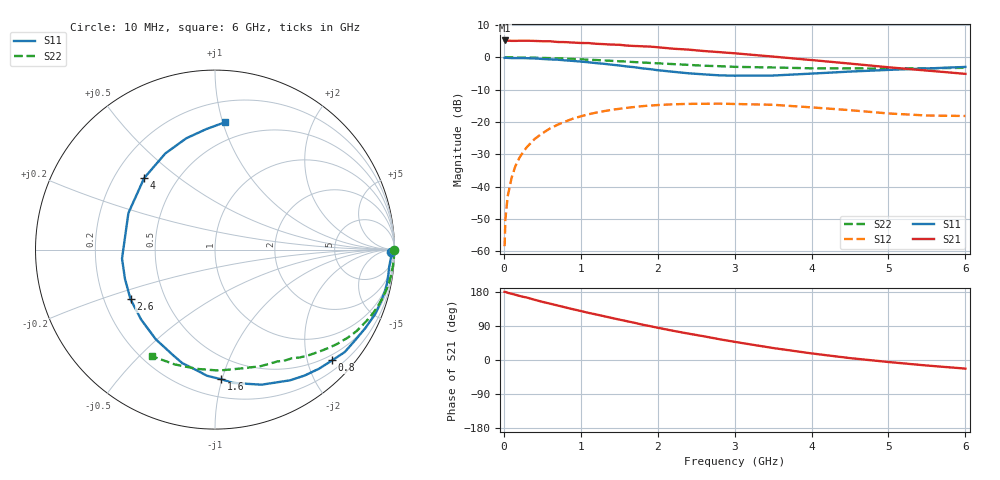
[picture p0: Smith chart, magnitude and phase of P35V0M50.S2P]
! SIEMENS Small Signal Semiconductors
! BFP181
! Si NPN RF Bipolar Junction Transistor in SOT143
! VCE = 5 V  IC = 0.5 mA
! Common Emitter S-Parameters:  March  1996
# GHz  S  MA  R  50
!  f  S11  S21  S12  S22
! GHz  MAG  ANG  MAG  ANG  MAG  ANG  MAG  ANG
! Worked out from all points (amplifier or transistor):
!   36 points, 10 MHz to 6 GHz, reference 50 ohm
!   highest |S21| = 5.2 dB at 10 MHz (marker M1)
!   |S21| within 3 dB of that: start of sweep to 2.476 GHz
!   unconditionally stable (mu >= 1): 3.793 GHz to end of sweep
!   at 250 MHz: K = 0.07, MSG = 17.2 dB, |S12| = -29.3 dB
!   at 1.4 GHz: K = 0.42, MSG = 10.1 dB, |S12| = -16.2 dB
!   at 6 GHz: K = 1.42, MAG = 2.6 dB, |S12| = -18.1 dB
!   S11 on the Smith chart (normalised r, x): 10 MHz: 69, -53; 800 MHz: 0.39, -2.46; 1.6 GHz: 0.33, -0.99; 2.6 GHz: 0.31, -0.25; 4 GHz: 0.33, +0.38; 6 GHz: 0.35, +1.02
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0.01  0.982 -0.8  1.827 179.8  0.0012 82.2  0.9999 -0.2
0.02  0.986 -1.2  1.825 179.7  0.0031 82.1  0.9998 -0.5
0.05  0.9817 -2.5  1.817 177.4  0.0071 91.5  0.998 -1.4
0.1  0.9753 -5.6  1.8 174.8  0.0136 84.0  0.9978 -2.6
0.15  0.9757 -8.3  1.799 172.2  0.0208 83.8  0.9966 -3.9
0.2  0.9765 -11.0  1.808 169.3  0.0276 81.9  0.9955 -5.3
0.3  0.97 -16.5  1.811 164.8  0.041 78.3  0.9924 -8.0
0.4  0.9628 -21.7  1.796 158.9  0.0546 74.4  0.9876 -10.6
0.6  0.9301 -32.8  1.776 148.7  0.0795 66.6  0.9737 -15.7
0.8  0.8982 -43.4  1.722 138.8  0.1019 59.3  0.955 -20.6
1.1  0.8399 -60.1  1.665 124.4  0.1315 48.6  0.9212 -27.5
1.5  0.7493 -82.4  1.567 106.7  0.16 35.9  0.8698 -35.9
1.6  0.7234 -87.2  1.522 102.4  0.1658 33.1  0.8598 -37.7
1.9  0.6581 -106.1  1.468 89.4  0.1796 24.6  0.8204 -43.2
2.2  0.5988 -123.4  1.362 77.1  0.188 17.2  0.7873 -48.3
2.6  0.546 -149.5  1.254 62.6  0.1915 8.4  0.7425 -54.6
3  0.5204 -174.5  1.156 47.9  0.1901 -0.1  0.7135 -60.9
3.5  0.5237 157.1  1.028 31.6  0.1848 -8.3  0.6974 -68.7
4  0.5609 134.7  0.909 17.4  0.1684 -14.4  0.6776 -77.9
4.5  0.6031 117.3  0.801 5.0  0.1525 -18.9  0.6743 -88.1
5.5  0.6733 94.1  0.625 -14.6  0.1261 -15.7  0.6778 -109.3
6  0.7112 85.6  0.556 -22.7  0.1239 -11.5  0.6898 -120.4
